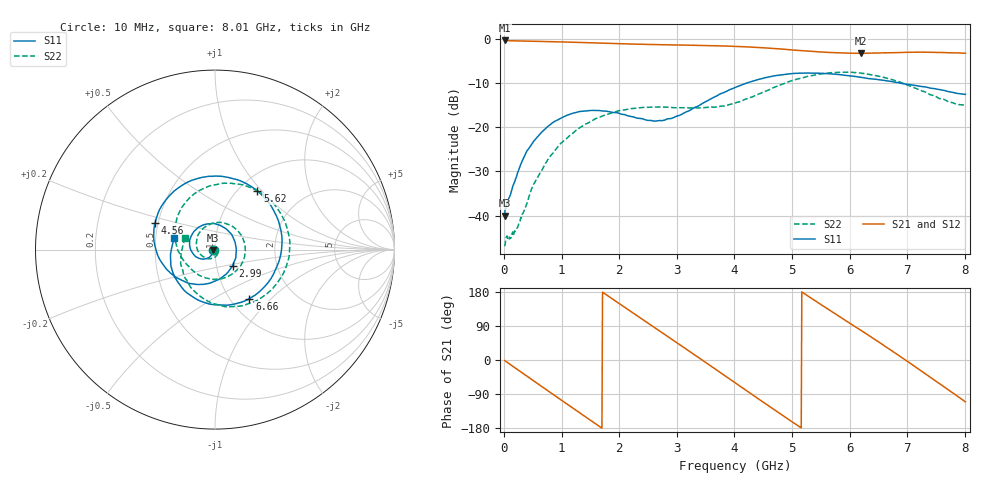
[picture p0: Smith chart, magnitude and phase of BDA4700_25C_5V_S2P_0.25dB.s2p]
!Agilent Technologies,E5071B,MY42404982,A.09.10
!Date: Mon Oct 20 13:26:05 2025
!Data & Calibration Information:
!Freq	S11:SOLT2(ON)	S21:SOLT2(ON)	S12:SOLT2(ON)	S22:SOLT2(ON)
# Hz S RI R 50
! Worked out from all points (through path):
!   801 points, 10 MHz to 8.01 GHz, reference 50 ohm
!   highest |S21| = -0.37 dB at 10 MHz (marker M1); lowest = -3.3 dB at 6.2 GHz (marker M2)
!   group delay of S21, straight-line fit = 286 ps
!   lowest |S11| = -40.0 dB at 10 MHz (marker M3), VSWR 1.02, Z = 49 - j0.242 ohm
!   |S11| at or under -10 dB: start of sweep to 4.213 GHz; 6.868 GHz to end of sweep
!   |S22| runs from -46.9 to -7.5 dB; largest |S21 - S12| = 0.0075
!   S11 on the Smith chart (normalised r, x): 10 MHz: 0.98, -0.00; 2.99 GHz: 1.20, -0.22; 4.56 GHz: 0.48, +0.16; 5.62 GHz: 1.21, +0.95; 6.66 GHz: 1.22, -0.75; 8.01 GHz: 0.63, +0.08
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1e7  -0.00967 -0.00247  0.9581 -0.0207  0.958 -0.0213  -0.00448 -0.000492
3.6e8  -0.0276 -0.039  0.7355 -0.5894  0.7355 -0.5898  0.0117 -0.000302
7.2e8  -0.0821 -0.0507  0.2123 -0.9069  0.2121 -0.9073  0.00404 -0.0388
1.02e9  -0.129 -0.0132  -0.2923 -0.8736  -0.2928 -0.8742  -0.0482 -0.0487
1.35e9  -0.1374 0.0626  -0.7279 -0.5438  -0.7285 -0.544  -0.1013 0.0105
1.63e9  -0.0956 0.1215  -0.8889 -0.1153  -0.8896 -0.1155  -0.0875 0.0931
1.92e9  -0.0206 0.145  -0.8148 0.3428  -0.8155 0.3433  -0.0037 0.1487
2.32e9  0.0793 0.0981  -0.3788 0.7819  -0.3782 0.7822  0.134 0.0965
2.68e9  0.1185 0.0044  0.1677 0.8428  0.168 0.8429  0.1642 -0.0412
2.99e9  0.0985 -0.0889  0.5845 0.6197  0.5833 0.6192  0.0949 -0.1362
3.49e9  -0.0374 -0.1891  0.8369 -0.0778  0.8369 -0.0779  -0.0698 -0.1511
4.01e9  -0.249 -0.13  0.4142 -0.711  0.4149 -0.7107  -0.1794 -0.0538
4.56e9  -0.3344 0.1482  -0.3644 -0.6974  -0.3647 -0.6984  -0.2209 0.1342
4.96e9  -0.1898 0.3536  -0.7028 -0.2694  -0.7041 -0.2716  -0.1185 0.308
5.35e9  0.0645 0.4039  -0.684 0.2286  -0.6848 0.2272  0.1154 0.3661
5.62e9  0.2363 0.3269  -0.495 0.499  -0.4952 0.5  0.2849 0.2945
6.2e9  0.3649 -0.034  0.1432 0.6693  0.1497 0.671  0.3999 -0.0854
6.66e9  0.1922 -0.2731  0.5911 0.3654  0.5924 0.3644  0.1908 -0.3005
6.68e9  0.181 -0.2792  0.6038 0.3444  0.6054 0.3433  0.1787 -0.3043
7.24e9  -0.1374 -0.2543  0.6213 -0.3374  0.6206 -0.3385  -0.1117 -0.234
7.63e9  -0.2449 -0.0938  0.2407 -0.6568  0.2396 -0.658  -0.1914 -0.0795
8.01e9  -0.2266 0.0633  -0.2391 -0.6436  -0.2384 -0.6453  -0.1655 0.0655
